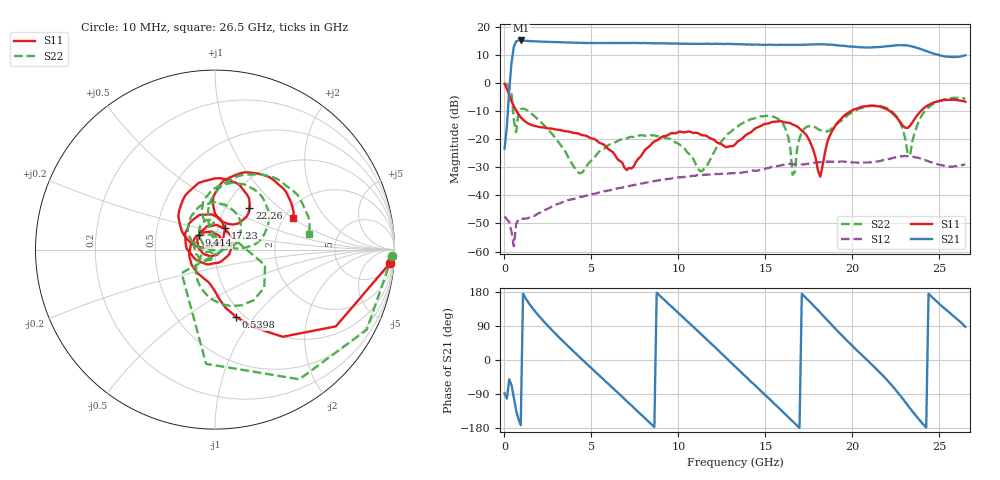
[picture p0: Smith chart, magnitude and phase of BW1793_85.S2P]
!Agilent Technologies,N5242A,MY52422126,A.09.90.01
!Agilent N5242A: A.09.90.01
!Date: Wednesday, September 07, 2016 21:52:28
!Correction: S11(Full 2 Port(1,2))
!S21(Full 2 Port(1,2))
!S12(Full 2 Port(1,2))
!S22(Full 2 Port(1,2))
!S2P File: Measurements: S11, S21, S12, S22:
# Hz S  dB  R 50
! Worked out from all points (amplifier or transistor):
!   201 points, 10 MHz to 26.5 GHz, reference 50 ohm
!   highest |S21| = 15.3 dB at 937.1 MHz (marker M1)
!   |S21| within 3 dB of that: 522.1 MHz to 23.91 GHz (23.38 GHz wide, 191 % of centre)
!   unconditionally stable (mu >= 1): start of sweep to end of sweep
!   at 4.381 GHz: K = 9.94, MAG = 14.5 dB, |S12| = -40.5 dB
!   at 13.26 GHz: K = 3.93, MAG = 14.1 dB, |S12| = -32.0 dB
!   at 26.5 GHz: K = 2.77, MAG = 12.2 dB, |S12| = -28.9 dB
!   S11 on the Smith chart (normalised r, x): 10 MHz: 7, -23; 539.8 MHz: 0.92, -0.82; 9.414 GHz: 0.83, +0.14; 17.23 GHz: 1.09, +0.26; 22.26 GHz: 1.29, +0.66; 26.5 GHz: 2.22, +1.01
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1e7  -0.20 -4.5  -23.25 -87.9  -47.49 0.2  -0.10 -2.1
2.749e8  -4.23 -52.2  -2.51 -50.9  -49.31 -19.4  -1.29 -56.9
5.398e8  -8.10 -72.5  13.05 -100.0  -58.09 32.7  -12.88 -144.9
9.3715e8  -12.15 -88.1  15.29 -172.0  -48.14 4.3  -9.21 -37.5
1.5994e9  -14.94 -105.1  15.01 137.7  -47.47 -6.6  -11.03 -92.3
2.3941e9  -15.94 -132.5  14.82 95.2  -44.98 -18.2  -15.72 -130.1
4.5133e9  -18.51 132.0  14.42 -1.0  -40.46 -81.4  -31.60 -118.8
6.76495e9  -28.24 -2.7  14.40 -96.8  -37.21 -152.2  -19.98 -151.7
8.88415e9  -19.90 160.5  14.27 171.6  -34.61 132.6  -18.85 135.4
9.41395e9  -18.43 136.9  14.22 148.8  -34.12 112.9  -19.67 119.3
1.11358e10  -17.80 62.9  14.08 75.6  -32.73 46.1  -30.47 108.7
1.3255e10  -21.84 -102.8  13.98 -16.7  -32.02 -36.0  -16.08 153.9
1.524175e10  -14.22 139.8  13.79 -103.1  -30.06 -110.5  -11.79 84.2
1.72285e10  -17.58 64.9  13.78 168.5  -28.91 161.7  -16.23 122.4
1.77583e10  -23.70 53.7  13.90 144.0  -28.39 140.3  -15.43 95.5
1.88179e10  -17.23 164.8  13.78 92.6  -27.99 92.6  -16.16 107.3
2.01424e10  -9.21 118.1  13.01 30.8  -28.23 36.2  -9.81 94.3
2.212915e10  -9.76 53.6  13.29 -59.8  -26.96 -42.5  -9.29 28.5
2.22616e10  -10.43 50.3  13.35 -66.5  -26.76 -48.9  -9.94 23.4
2.30563e10  -15.89 63.4  13.57 -111.7  -25.92 -93.0  -20.25 5.3
2.3851e10  -10.52 91.5  12.40 -158.0  -26.66 -139.9  -13.01 99.9
2.65e10  -6.57 22.2  9.98 87.2  -28.89 109.1  -5.48 9.4
